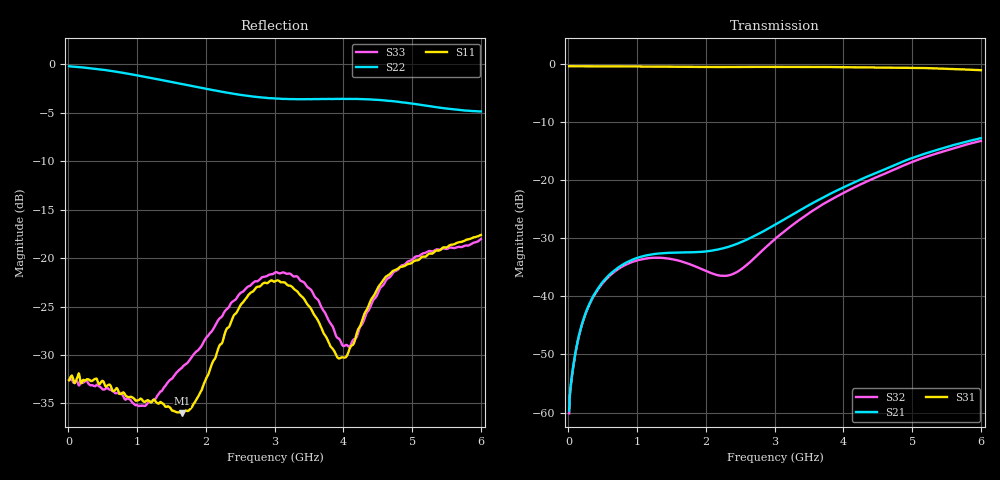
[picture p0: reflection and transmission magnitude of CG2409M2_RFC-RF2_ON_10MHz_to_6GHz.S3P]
!CEL
!CG2409M2
!Port1: RFC Port2: RF1  Port3: RF2
!Freq	S11 S12	S13 S21 S22 S23 S31 S32 S33
# Hz S dB R 50
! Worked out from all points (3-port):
!   600 points, 10 MHz to 6 GHz, reference 50 ohm
!   strongest paths, dB at 10 MHz, 1.51 GHz, 3.01 GHz, 4.51 GHz, 6 GHz:
!     S31: -0.3, -0.4, -0.5, -0.6, -1.0
!     S21: -59.7, -32.5, -27.6, -18.5, -12.7
!     S32: -60.1, -33.6, -30.1, -19.3, -13.2
!   lowest |S11| = -36.0 dB at 1.65 GHz (marker M1), VSWR 1.03, Z = 51.5 - j0.564 ohm
!   |S11| at or under -10 dB: start of sweep to end of sweep
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1e7  -32.61 -2.6  -59.69 45.7  -0.34 -0.3
     -59.66 45.8  -0.18 -1.1  -60.15 45.9
     -0.34 -0.3  -60.14 45.8  -32.55 -3.9
1.9e8  -32.92 3.3  -45.06 70.2  -0.36 -2.9
       -45.05 70.3  -0.30 -14.3  -45.18 66.8
       -0.36 -2.9  -45.16 66.8  -32.68 4.5
4.9e8  -32.67 4.7  -37.67 68.7  -0.37 -6.9
       -37.65 68.9  -0.54 -35.6  -37.84 58.1
       -0.37 -6.9  -37.85 58.0  -33.50 11.1
1.03e9  -34.63 -20.9  -33.24 58.9  -0.40 -13.5
        -33.25 59.0  -1.18 -71.3  -33.70 31.9
        -0.39 -13.6  -33.70 31.8  -35.27 -6.5
1.65e9  -36.02 -20.3  -32.43 59.3  -0.46 -20.7
        -32.44 59.2  -2.03 -107.7  -33.99 -4.5
        -0.45 -20.8  -34.00 -4.5  -31.32 -15.4
2.34e9  -27.06 29.5  -31.42 79.5  -0.48 -28.7
        -31.41 79.4  -2.95 -145.4  -36.30 -81.4
        -0.48 -28.7  -36.35 -81.3  -24.98 28.2
3.01e9  -22.38 34.7  -27.66 98.2  -0.45 -36.4
        -27.62 97.9  -3.53 179.8  -30.05 -156.1
        -0.45 -36.5  -30.06 -155.9  -21.47 38.6
4.01e9  -30.27 93.5  -21.18 99.9  -0.51 -49.2
        -21.16 99.8  -3.56 143.8  -22.14 158.9
        -0.50 -49.4  -22.12 158.9  -29.07 -23.4
4.62e9  -21.90 146.3  -18.00 93.2  -0.59 -57.9
        -18.02 92.8  -3.74 128.7  -18.77 141.8
        -0.59 -58.0  -18.76 142.1  -22.29 -101.2
6e9  -17.61 146.2  -12.86 65.1  -1.04 -79.5
     -12.74 65.2  -4.86 84.1  -13.22 104.3
     -1.03 -79.8  -13.22 104.8  -18.03 -141.2
